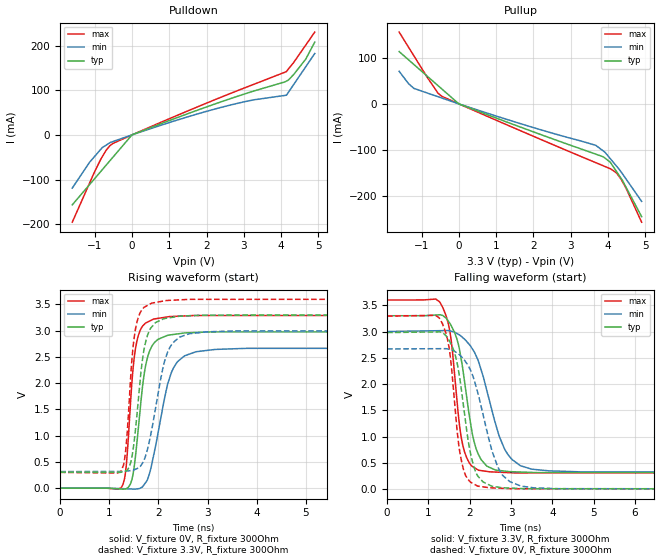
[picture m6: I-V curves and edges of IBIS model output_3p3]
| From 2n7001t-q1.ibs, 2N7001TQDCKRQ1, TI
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|   output_3p3 Model
[Model]   output_3p3
Model_type   Output
Polarity   Non-Inverting
Vmeas = 1.65
Vref = 0
Cref = 2pF
Rref = 100000
|   typ   min   max
C_comp   1.158pF   0.790pF   1.411pF
|  Where Nom  PVT is Nominal Process,   3.3V,  27C
|   Fast PVT is Strong Process,   3.6V, -40C
|   Slow PVT is Weak Process,   3V, 130C
[Voltage Range]   3.3   3   3.6
|Junction Temperature
[Temperature Range]   27   130   -40
[Pullup Reference]   3.3   3   3.6
[Pulldown Reference]   0   -0   -0
[Power Clamp Reference]   3.3   3   3.6
[GND Clamp Reference]   0   0   0
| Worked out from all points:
|   slope of the pulldown table from 0 to 0.495 V, typ, clamps not added: 30.9 ohm
|   slope of the pullup table from 0 to 0.495 V, typ, clamps not added: 32.2 ohm
|   falling waveform, V_fixture 3.3V, R_fixture 300Ohm: 20-80 % time 364ps typ, 599ps min, 268ps max; typ from 3.3 V to 0.307 V
|   rising waveform, V_fixture 0V, R_fixture 300Ohm: 20-80 % time 220ps typ, 358ps min, 164ps max; typ from 0 V to 2.98 V
|   rising waveform, V_fixture 3.3V, R_fixture 300Ohm: 20-80 % time 212ps typ, 334ps min, 162ps max; typ from 0.307 V to 3.3 V
|   falling waveform, V_fixture 0V, R_fixture 300Ohm: 20-80 % time 343ps typ, 543ps min, 259ps max; typ from 2.98 V to 0 V
[Pulldown]
|   Voltage   I(typ)   I(min)   I(max)
-1.6V     -156.6mA   -119mA     -195.4mA
-1.136V   -111.2mA   -61.27mA   -107.9mA
-829.7mV  -81.21mA   -31.66mA   -53.62mA
-601.8mV  -58.9mA    -18.14mA   -25.04mA
-513.4mV  -50.25mA   -15.02mA   -19.27mA
-28.17uV  -915.7nA   -802nA     -1.032uA
2.346V    72.75mA    60.61mA    82.9mA
3.275V    98.46mA    78.6mA     113.5mA
4.141V    120.4mA    88.82mA    142mA
4.34V     135.6mA    113.3mA    162.7mA
4.658V    169.5mA    152.5mA    201mA
4.9V      207.7mA    182.2mA    230.1mA
[Pullup]
|   Voltage   I(typ)   I(min)   I(max)
-1.6V     114mA      70.98mA    156.5mA
-1.203V   85.73mA    33.67mA    104.5mA
-557mV    39.69mA    15.59mA    23.19mA
-458.4mV  32.66mA    12.83mA    16.54mA
-28.17uV  845.5nA    815.1nA    1.012uA
3.671V    -109.6mA   -90.4mA    -128.2mA
3.87V     -115.3mA   -102.5mA   -135mA
4.057V    -126.9mA   -119.1mA   -141.3mA
4.228V    -147.7mA   -135.8mA   -150.7mA
4.344V    -161.8mA   -147.7mA   -163.6mA
4.483V    -181.8mA   -163.9mA   -183.9mA
4.9V      -246mA     -212.6mA   -258mA
[Ramp]
R_load = 300
|   typ   min   max
dV/dt_r   1.7882/2.19429e-10   1.60117/3.5333e-10   1.97555/1.63828e-10
dV/dt_f   1.7957/3.63649e-10   1.61014/5.93106e-10   1.9792/2.68075e-10
[Falling Waveform]
V_fixture = 3.3V
V_fixture_min = 3V
V_fixture_max = 3.6V
R_fixture = 300Ohm
C_fixture = 0F
|   Time   V(typ)   V(min)   V(max)
0s        3.3V       3V         3.6V
1.288ns   3.319V     3.016V     3.546V
1.523ns   3.153V     3.012V     2.992V
1.763ns   2.617V     2.931V     1.161V
1.878ns   2.035V     2.852V     703.2mV
2.154ns   776.4mV    2.541V     389.6mV
2.483ns   414.2mV    1.67V      330.3mV
3.003ns   332.6mV    583.4mV    312.4mV
3.915ns   315.3mV    348.8mV    309.6mV
40ns      307.2mV    316.4mV    301.3mV
[Rising Waveform]
V_fixture = 0V
V_fixture_min = 0V
V_fixture_max = 0V
R_fixture = 300Ohm
C_fixture = 0F
|   Time   V(typ)   V(min)   V(max)
0s        -44.38nV   149.9nV    -35.69nV
1.243ns   -15.83mV   -8.402mV   10.07mV
1.344ns   -10.75mV   -11.86mV   412.5mV
1.458ns   154.4mV    -15.78mV   1.984V
1.592ns   1.143V     -9.754mV   2.908V
1.795ns   2.542V     210mV      3.17V
2.223ns   2.915V     2.082V     3.266V
2.533ns   2.955V     2.52V      3.279V
3.792ns   2.975V     2.662V     3.287V
40ns      2.98V      2.669V     3.293V
[Rising Waveform]
V_fixture = 3.3V
V_fixture_min = 3V
V_fixture_max = 3.6V
R_fixture = 300Ohm
C_fixture = 0F
|   Time   V(typ)   V(min)   V(max)
0s        307.2mV    316.4mV    301.3mV
1.236ns   303.2mV    317.5mV    318.3mV
1.333ns   325mV      322.9mV    711.5mV
1.438ns   493.8mV    334.9mV    2.157V
1.567ns   1.437V     374.1mV    3.176V
1.76ns    2.857V     682.5mV    3.47V
2.161ns   3.235V     2.521V     3.573V
2.43ns    3.274V     2.875V     3.585V
3.554ns   3.294V     2.993V     3.594V
40ns      3.3V       3V         3.6V
[Falling Waveform]
|Gnd
V_fixture = 0V
V_fixture_min = 0V
V_fixture_max = 0V
R_fixture = 300Ohm
C_fixture = 0F
|   Time   V(typ)   V(min)   V(max)
0s        2.98V      2.669V     3.293V
1.278ns   2.993V     2.673V     3.242V
1.498ns   2.835V     2.662V     2.708V
1.729ns   2.262V     2.576V     881.6mV
1.849ns   1.594V     2.481V     378.1mV
2.134ns   348.6mV    2.008V     83.56mV
2.483ns   76.59mV    899mV      26.36mV
2.971ns   21.18mV    143.5mV    9.502mV
4.137ns   8.49mV     8.855mV    7.994mV
40ns      7.923nV    182nV      18.71nV
